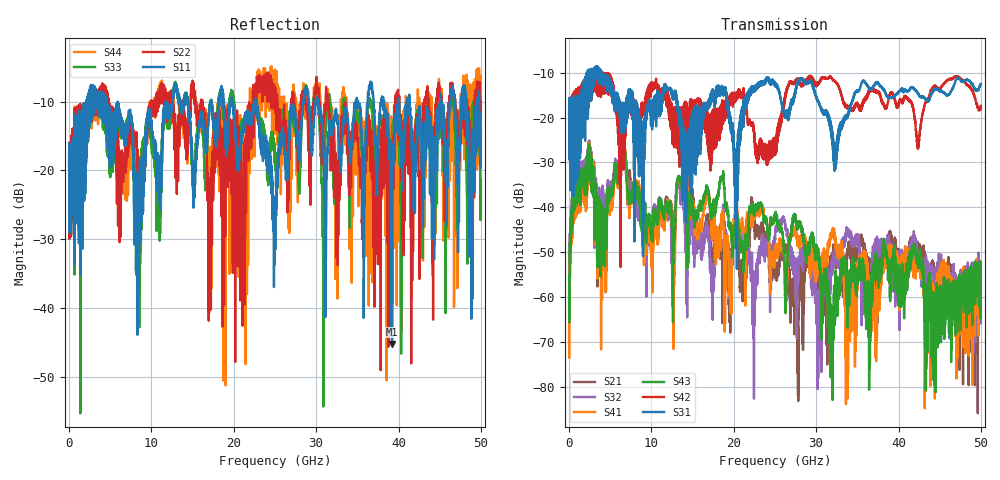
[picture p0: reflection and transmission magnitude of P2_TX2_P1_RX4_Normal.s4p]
!Keysight Technologies,N5225B,MY57041031,A.13.20.10
!Date: Friday, May 31, 2019 11:19:48
!Correction: S11(Full 4 Port(1,2,3,4))
!S12(Full 4 Port(1,2,3,4))
!S13(Full 4 Port(1,2,3,4))
!S14(Full 4 Port(1,2,3,4))
!S21(Full 4 Port(1,2,3,4))
!S22(Full 4 Port(1,2,3,4))
!S23(Full 4 Port(1,2,3,4))
!S24(Full 4 Port(1,2,3,4))
!S31(Full 4 Port(1,2,3,4))
!S32(Full 4 Port(1,2,3,4))
!S33(Full 4 Port(1,2,3,4))
!S34(Full 4 Port(1,2,3,4))
!S41(Full 4 Port(1,2,3,4))
!S42(Full 4 Port(1,2,3,4))
!S43(Full 4 Port(1,2,3,4))
!S44(Full 4 Port(1,2,3,4))
!S4P File: Measurements: <S11,S12,S13,S14>,
!<S21,S22,S23,S24>,
!<S31,S32,S33,S34>,
!<S41,S42,S43,S44>:
# Hz S  dB  R 50.0
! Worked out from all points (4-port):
!   5000 points, 10 MHz to 50 GHz, reference 50 ohm
!   strongest paths, dB at 10 MHz, 12.51 GHz, 25.01 GHz, 37.51 GHz, 50 GHz:
!     S31: -19.3, -14.8, -13.0, -12.4, -12.6
!     S42: -19.5, -19.3, -25.6, -14.5, -17.4
!     S43: -57.6, -43.1, -42.0, -52.5, -56.2
!     S41: -65.5, -43.1, -50.2, -56.0, -55.2
!     S32: -60.4, -52.2, -46.9, -48.4, -58.6
!     S21: -62.2, -43.9, -54.3, -57.8, -60.1
!   lowest |S11| = -45.2 dB at 39.22 GHz (marker M1), VSWR 1.01, Z = 49.9 + j0.528 ohm
!   |S11| at or under -10 dB: 4.481 GHz to 11.72 GHz (7.238 GHz wide, 89.4 % of centre); 22.73 GHz to 28.43 GHz (5.704 GHz wide, 22.3 % of centre); 30.26 GHz to 34.82 GHz (4.559 GHz wide, 14 % of centre)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
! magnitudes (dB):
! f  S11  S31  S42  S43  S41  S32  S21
! 10 MHz  -19.2  -19.3  -19.5  -57.6  -65.5  -60.4  -62.2
! 6.64 GHz  -14.0  -21.2  -25.6  -27.2  -27.1  -27.6  -26.9
! 19.47 GHz  -11.5  -20.3  -15.7  -44.6  -55.4  -54.7  -61.9
! 31.92 GHz  -13.7  -23.2  -11.4  -67.2  -45.5  -53.5  -51.6
! 33.81 GHz  -12.9  -19.7  -17.8  -57.5  -82.4  -45.2  -49.6
! 39.22 GHz  -45.2  -15.7  -14.6  -52.5  -51.0  -51.6  -48.0
! 50 GHz  -14.0  -12.6  -17.4  -56.2  -55.2  -58.6  -60.1
